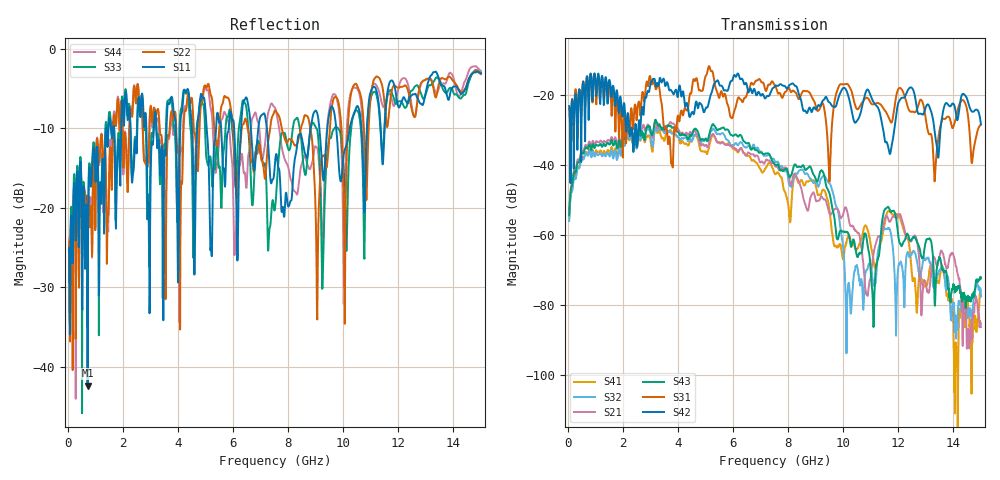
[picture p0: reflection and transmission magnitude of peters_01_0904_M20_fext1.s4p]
# MHZ S RI R 50.00
! FREQ  S11  S12  S13  S14
!  S21  S22  S23  S24
!  S31  S32  S33  S34
!  S41  S42  S43  S44
!  REAL  IMAG  REAL  IMAG  REAL  IMAG  REAL  IMAG
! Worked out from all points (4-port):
!   1496 points, 50 MHz to 15 GHz, reference 50 ohm
!   strongest paths, dB at 50 MHz, 3.79 GHz, 7.53 GHz, 11.27 GHz, 15 GHz:
!     S42: -23.1, -19.1, -17.4, -23.7, -28.3
!     S31: -23.8, -39.4, -17.2, -22.2, -28.4
!     S43: -54.4, -29.4, -39.9, -66.4, -72.3
!     S21: -53.7, -28.1, -40.3, -60.4, -86.3
!     S32: -56.0, -31.1, -39.0, -64.4, -77.6
!     S41: -55.8, -30.8, -42.6, -65.9, -77.5
!   lowest |S11| = -42.4 dB at 720 MHz (marker M1), VSWR 1.02, Z = 49.7 - j0.713 ohm
!   |S11| at or under -10 dB: start of sweep to 1.385 GHz; 7.23 GHz to 8.818 GHz (1.588 GHz wide, 19.8 % of centre); 9.748 GHz to 10.24 GHz (490.5 MHz wide, 4.91 % of centre)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
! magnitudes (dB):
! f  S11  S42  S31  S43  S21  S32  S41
! 50 MHz  -25.1  -23.1  -23.8  -54.4  -53.7  -56.0  -55.8
! 720 MHz  -42.4  -16.0  -15.0  -35.4  -34.7  -37.3  -36.9
! 3.77 GHz  -6.1  -18.8  -39.7  -29.2  -28.0  -30.9  -30.5
! 5.3 GHz  -12.9  -17.0  -15.0  -28.5  -31.3  -29.7  -31.2
! 9.35 GHz  -13.8  -20.7  -25.8  -44.7  -49.9  -43.4  -47.7
! 10.28 GHz  -9.4  -23.3  -18.4  -63.2  -57.5  -82.5  -62.1
! 15 GHz  -3.1  -28.3  -28.4  -72.3  -86.3  -77.6  -77.5
